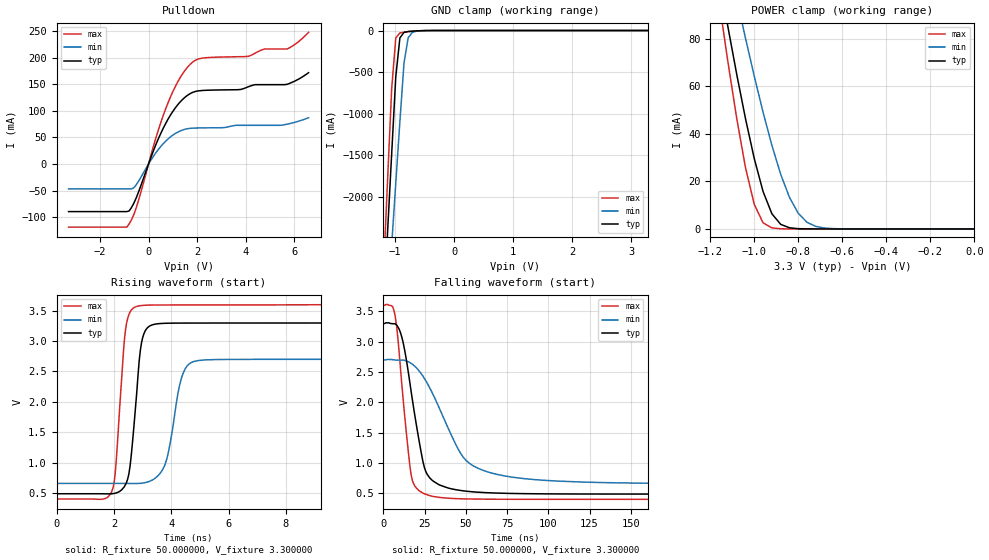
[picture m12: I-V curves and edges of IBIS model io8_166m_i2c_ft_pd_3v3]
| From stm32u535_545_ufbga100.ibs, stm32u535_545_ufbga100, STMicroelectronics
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|   Model io8_166m_i2c_ft_pd_3v3
[Model]  io8_166m_i2c_ft_pd_3v3
Model_type I/O_open_drain
Polarity   Non-Inverting
Enable   Active-Low
Vinl =   0.990000V
Vinh =   2.310000V
Vmeas =  1.600000V
Cref =   50.000000pF
Rref =   1.000000
Vref =   1.650000V
C_comp   3.523800pF   3.496000pF   3.564000pF
[Temperature Range]   25.000000   0.140000k   -40.000000
[Pullup Reference]   3.300000V   2.700000V   3.600000V
[Pulldown Reference]   0.0V   0.0V   0.0V
[POWER Clamp Reference]   3.300000V   2.700000V   3.600000V
[GND Clamp Reference]   0.0V   0.0V   0.0V
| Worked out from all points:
|   slope of the pulldown table from 0 to 0.495 V, typ, clamps not added: 8.73 ohm
|   GND clamp passes 1 mA (typ) near -0.50 V on its own axis
|   POWER clamp passes 1 mA (typ) near -0.85 V on its own axis
|   rising waveform, R_fixture 50.000000, V_fixture 3.300000: 20-80 % time 308ps typ, 455ps min, 273ps max; typ from 0.49 V to 3.3 V
|   falling waveform, R_fixture 50.000000, V_fixture 3.300000: 20-80 % time 10.1ns typ, 22.3ns min, 6.6ns max; typ from 3.3 V to 0.49 V
[Pulldown]
|Voltage   I(typ)   I(min)   I(max)
-3.3V     -89.72mA   -47.06mA   -119mA
-900mV    -89.72mA   -47.06mA   -119mA
-500mV    -62.92mA   -38.71mA   -81.44mA
300mV     36.2mA     21.01mA    48.7mA
800mV     84.07mA    46.96mA    114.9mA
1.3V      116.7mA    62.09mA    162.4mA
1.8V      134.4mA    67.39mA    191.2mA
2.3V      138.6mA    67.98mA    199.8mA
4.1V      145.1mA    72.78mA    202.7mA
4.8V      149.4mA    72.78mA    216.5mA
5.7V      149.8mA    74.8mA     216.5mA
6.6V      171.9mA    87.1mA     247.9mA
[GND_clamp]
|Voltage   I(typ)   I(min)   I(max)
-3.3V     -9.098A    -9.372A    -9.671A
-1.2V     -3.386A    -4.091A    -2.933A
-1.13V    -2.437A    -3.34A     -1.815A
-1.06V    -1.49A     -2.588A    -705.6mA
-990mV    -555.7mA   -1.839A    -89.05mA
-920mV    -88.14mA   -1.093A    -28.79mA
-850mV    -22.37mA   -387.4mA   -19.86mA
-780mV    -12.13mA   -88.01mA   -13.89mA
-710mV    -7.72mA    -22.53mA   -8.86mA
-640mV    -4.556mA   -7.872mA   -4.884mA
-360mV    -39.7uA    -179.9uA   -19.45uA
3.28V     83.52uA    56.87uA    102.4uA
[POWER_clamp]
|Voltage   I(typ)   I(min)   I(max)
-3.28V    1.355A     1.167A     1.664A
-1.16V    105.7mA    131.6mA    95.69mA
-1.12V    84.97mA    114mA      70.27mA
-1.08V    65.05mA    96.83mA    46.54mA
-1.04V    46.34mA    80.15mA    25.76mA
-1V       29.51mA    64.13mA    10.3mA
-960mV    15.69mA    48.99mA    2.571mA
-920mV    6.373mA    35.1mA     455.6uA
-840mV    490.7uA    13.24mA    11.36uA
-760mV    27.33uA    2.767mA    278.2nA
-640mV    347.6nA    134.1uA    16.76nA
0V        0A         19.95nA    0A
[Ramp]
| variable   typ   min   max
dV/dt_r  1.68577/0.50485n   1.22392/0.57526n   1.91752/0.30506n
dV/dt_f  1.68577/10.07580n   1.22392/22.28016n   1.91752/6.57429n
R_load = 50.000000
[Rising Waveform]
R_fixture= 50.000000
V_fixture= 3.300000
V_fixture_min= 2.700000
V_fixture_max= 3.600000
|time   V(typ)   V(min)   V(max)
0s        489.8mV    659.5mV    403.4mV
1.922ns   489.5mV    659.5mV    523.4mV
2.042ns   498.3mV    659.5mV    804.6mV
2.402ns   639.4mV    659.3mV    3.172V
2.803ns   2.186V     658.6mV    3.569V
3.163ns   3.214V     681.3mV    3.589V
3.764ns   3.29V      946.6mV    3.591V
4.364ns   3.294V     2.401V     3.592V
4.845ns   3.294V     2.67V      3.592V
19.94ns   3.299V     2.699V     3.599V
[Falling Waveform]
R_fixture= 50.000000
V_fixture= 3.300000
V_fixture_min= 2.700000
V_fixture_max= 3.600000
|time   V(typ)   V(min)   V(max)
0s        3.299V     2.699V     3.599V
5.606ns   3.296V     2.704V     3.578V
7.207ns   3.295V     2.698V     3.413V
12.01ns   2.979V     2.696V     2.042V
17.62ns   2.035V     2.628V     708.6mV
24.02ns   1.02V      2.43V      505.2mV
28.83ns   736.9mV    2.2V       459mV
49.65ns   539.5mV    1.059V     410.4mV
76.88ns   500.8mV    774mV      404.3mV
398.8ns   489.8mV    659.5mV    403.4mV
